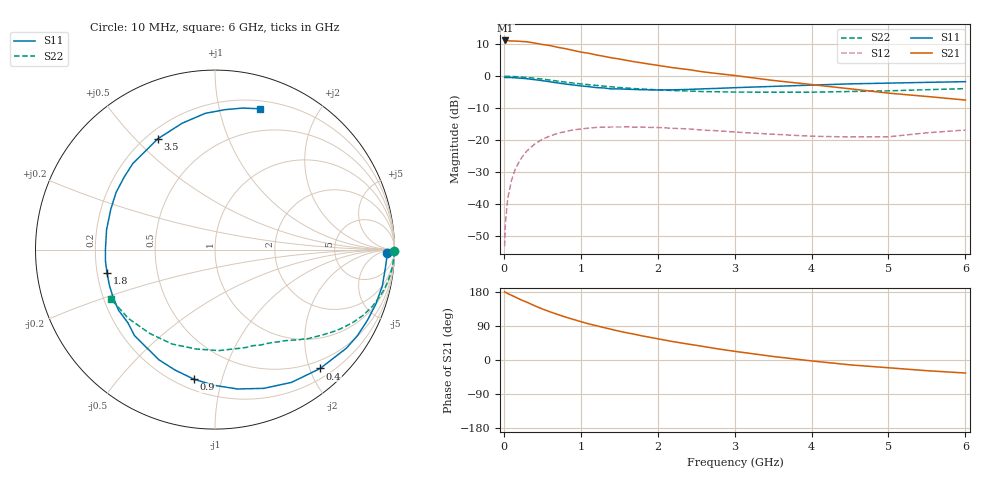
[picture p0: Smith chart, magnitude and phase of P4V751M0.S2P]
! SIEMENS Small Signal Semiconductors
! BFP182
! Si NPN RF Bipolar Junction Transistor in SOT143
! VCE = 0.75 V  IC = 1 mA
! Common Emitter S-Parameters:  March  1996
# GHz  S  MA  R  50
!  f  S11  S21  S12  S22
! GHz  MAG  ANG  MAG  ANG  MAG  ANG  MAG  ANG
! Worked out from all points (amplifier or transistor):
!   36 points, 10 MHz to 6 GHz, reference 50 ohm
!   highest |S21| = 11.2 dB at 20 MHz (marker M1)
!   |S21| within 3 dB of that: start of sweep to 881.3 MHz
!   unconditionally stable (mu >= 1): 2.5 GHz to end of sweep
!   at 250 MHz: K = 0.10, MSG = 17.9 dB, |S12| = -24.9 dB
!   at 1.4 GHz: K = 0.58, MSG = 10.8 dB, |S12| = -15.9 dB
!   at 6 GHz: K = 1.26, MAG = 1.6 dB, |S12| = -16.8 dB
!   S11 on the Smith chart (normalised r, x): 10 MHz: 39, -21; 400 MHz: 0.36, -2.17; 900 MHz: 0.26, -0.82; 1.8 GHz: 0.24, -0.10; 3.5 GHz: 0.24, +0.58; 6 GHz: 0.27, +1.33
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0.01  0.9611 -1.2  3.585 179.4  0.0022 89.9  0.9968 -0.5
0.02  0.9582 -2.7  3.633 178.8  0.0049 88.2  0.9977 -1.1
0.05  0.9547 -6.1  3.606 175.3  0.0121 86.9  0.9964 -2.6
0.1  0.9541 -12.3  3.563 170.7  0.0238 82.5  0.9936 -5.2
0.15  0.9461 -18.7  3.549 165.9  0.0355 77.9  0.987 -7.9
0.2  0.9363 -24.8  3.531 161.0  0.0466 74.7  0.9791 -10.4
0.3  0.9152 -36.9  3.466 152.5  0.0681 66.7  0.958 -15.3
0.4  0.8843 -48.5  3.307 143.1  0.0867 59.7  0.9323 -19.8
0.5  0.854 -60.0  3.144 134.8  0.1032 53.0  0.903 -23.9
0.6  0.8196 -70.6  3.024 127.2  0.1167 47.2  0.8712 -27.6
0.8  0.7564 -90.2  2.702 113.4  0.1364 36.3  0.8103 -34.0
0.9  0.732 -99.1  2.543 107.3  0.1448 31.7  0.7845 -36.4
1.1  0.6889 -117.0  2.294 95.5  0.1546 23.7  0.7385 -41.2
1.3  0.6564 -133.1  2.052 85.6  0.1601 16.7  0.7004 -45.3
1.5  0.6347 -147.8  1.864 76.0  0.1608 11.0  0.6666 -49.1
1.8  0.6154 -167.9  1.615 63.6  0.1607 4.5  0.6322 -53.8
2.2  0.6143 169.6  1.36 48.5  0.1535 -2.9  0.5985 -60.9
2.8  0.648 141.2  1.095 28.8  0.1401 -9.5  0.5723 -72.2
3.5  0.6946 117.3  0.861 9.3  0.124 -11.4  0.563 -87.9
4.5  0.761 94.1  0.637 -12.8  0.1123 -5.2  0.5778 -114.4
5.5  0.8033 79.0  0.483 -28.2  0.1306 5.2  0.6166 -141.5
6  0.8231 72.4  0.425 -34.4  0.1444 4.9  0.6405 -154.3
